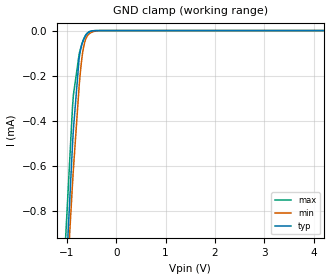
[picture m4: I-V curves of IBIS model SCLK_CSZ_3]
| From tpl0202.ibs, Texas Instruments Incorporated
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[Model]   SCLK_CSZ_3
Model_type   Input
Vinl = .8
Vinh = 2.1
|   typ   min   max
C_comp   2.500e-15   2.500e-15   2.500e-15
[Voltage Range]   3   2.7   3.3
[Temperature Range]   27   85   -40
[Power Clamp Reference]   3   2.7   3.3
[GND Clamp Reference]   -0   -0   -0
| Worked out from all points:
|   GND clamp passes 1 mA (typ) near -1.00 V on its own axis
[GND Clamp]
|   Voltage   I(typ)   I(min)   I(max)
-3V       -13.25mA   -11.89mA   -15.29mA
-1.038V   -1.183mA   -1.271mA   -981.2uA
-885mV    -508.9uA   -681.7uA   -341.4uA
-867mV    -440.7uA   -617.1uA   -287.4uA
-750mV    -122.5uA   -246.2uA   -104.7uA
-696mV    -63uA      -125.7uA   -60.37uA
-660mV    -40.36uA   -73.23uA   -38.2uA
-633mV    -28.14uA   -48uA      -25.62uA
-588mV    -14.12uA   -24.6uA    -11.65uA
-534mV    -5.067uA   -12.06uA   -3.714uA
-282mV    0A         -2.34nA    0A
5.991V    0A         0A         0A
[POWER Clamp]
|   Voltage   I(typ)   I(min)   I(max)
-3V       0A         0A         0A
0V        0A         0A         0A
6V        0A         0A         0A
